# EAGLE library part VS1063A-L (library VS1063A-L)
VS1063 - MP3 / Ogg Vorbis Encoder and Audio Codec Circuit, LQFP48 7x7x1.4mm Source: Datasheet
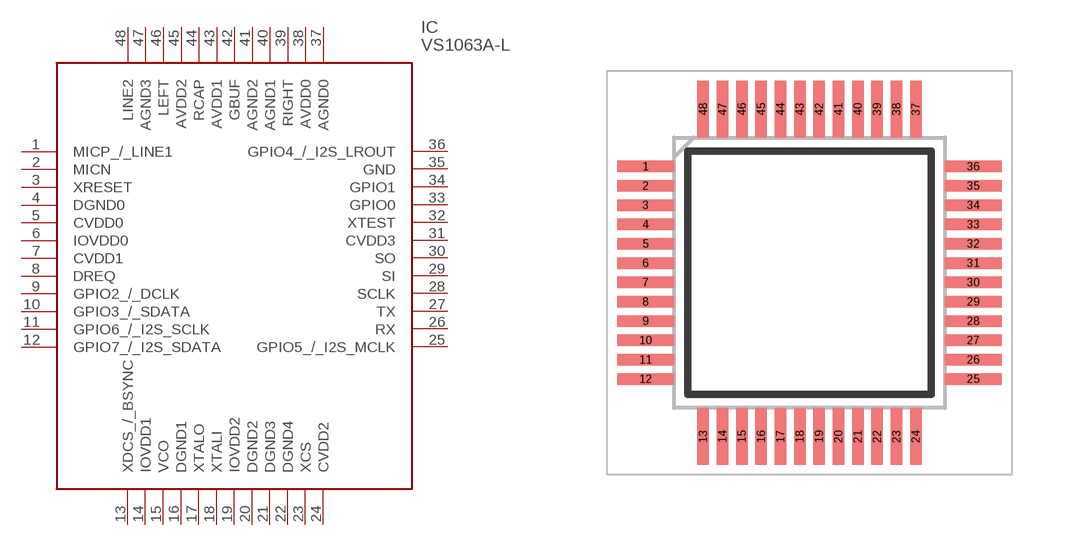
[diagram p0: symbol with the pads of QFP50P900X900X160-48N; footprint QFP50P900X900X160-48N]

Designator prefix IC

## VS1063A-L (Description: VS1063 - MP3 / Ogg Vorbis Encoder and Audio Codec Circuit, LQFP48 7x7x1.4mm; Height: 1.6mm; Manufacturer_Name: VLSI; Manufacturer_Part_Number: VS1063A-L)  [QFP50P900X900X160-48N]
1  MICP_/_LINE1
2  MICN
3  XRESET
4  DGND0
5  CVDD0
6  IOVDD0
7  CVDD1
8  DREQ
9  GPIO2_/_DCLK
10  GPIO3_/_SDATA
11  GPIO6_/_I2S_SCLK
12  GPIO7_/_I2S_SDATA
13  XDCS_/_BSYNC
14  IOVDD1
15  VCO
16  DGND1
17  XTALO
18  XTALI
19  IOVDD2
20  DGND2
21  DGND3
22  DGND4
23  XCS
24  CVDD2
25  GPIO5_/_I2S_MCLK
26  RX
27  TX
28  SCLK
29  SI
30  SO
31  CVDD3
32  XTEST
33  GPIO0
34  GPIO1
35  GND
36  GPIO4_/_I2S_LROUT
37  AGND0
38  AVDD0
39  RIGHT
40  AGND1
41  AGND2
42  GBUF
43  AVDD1
44  RCAP
45  AVDD2
46  LEFT
47  AGND3
48  LINE2

## Footprint QFP50P900X900X160-48N (pad centres in mm)
QFP 7x7x1.4
smd 1.475 x 0.3: 1 -4.238,2.75; 2 -4.238,2.25; 3 -4.238,1.75; 4 -4.238,1.25; 5 -4.238,0.75; 6 -4.238,0.25; 7 -4.238,-0.25; 8 -4.238,-0.75; 9 -4.238,-1.25; 10 -4.238,-1.75; 11 -4.238,-2.25; 12 -4.238,-2.75; 25 4.238,-2.75; 26 4.238,-2.25; 27 4.238,-1.75; 28 4.238,-1.25; 29 4.238,-0.75; 30 4.238,-0.25; 31 4.238,0.25; 32 4.238,0.75; 33 4.238,1.25; 34 4.238,1.75; 35 4.238,2.25; 36 4.238,2.75
smd 0.3 x 1.475: 13 -2.75,-4.238; 14 -2.25,-4.238; 15 -1.75,-4.238; 16 -1.25,-4.238; 17 -0.75,-4.238; 18 -0.25,-4.238; 19 0.25,-4.238; 20 0.75,-4.238; 21 1.25,-4.238; 22 1.75,-4.238; 23 2.25,-4.238; 24 2.75,-4.238; 37 2.75,4.238; 38 2.25,4.238; 39 1.75,4.238; 40 1.25,4.238; 41 0.75,4.238; 42 0.25,4.238; 43 -0.25,4.238; 44 -0.75,4.238; 45 -1.25,4.238; 46 -1.75,4.238; 47 -2.25,4.238; 48 -2.75,4.238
